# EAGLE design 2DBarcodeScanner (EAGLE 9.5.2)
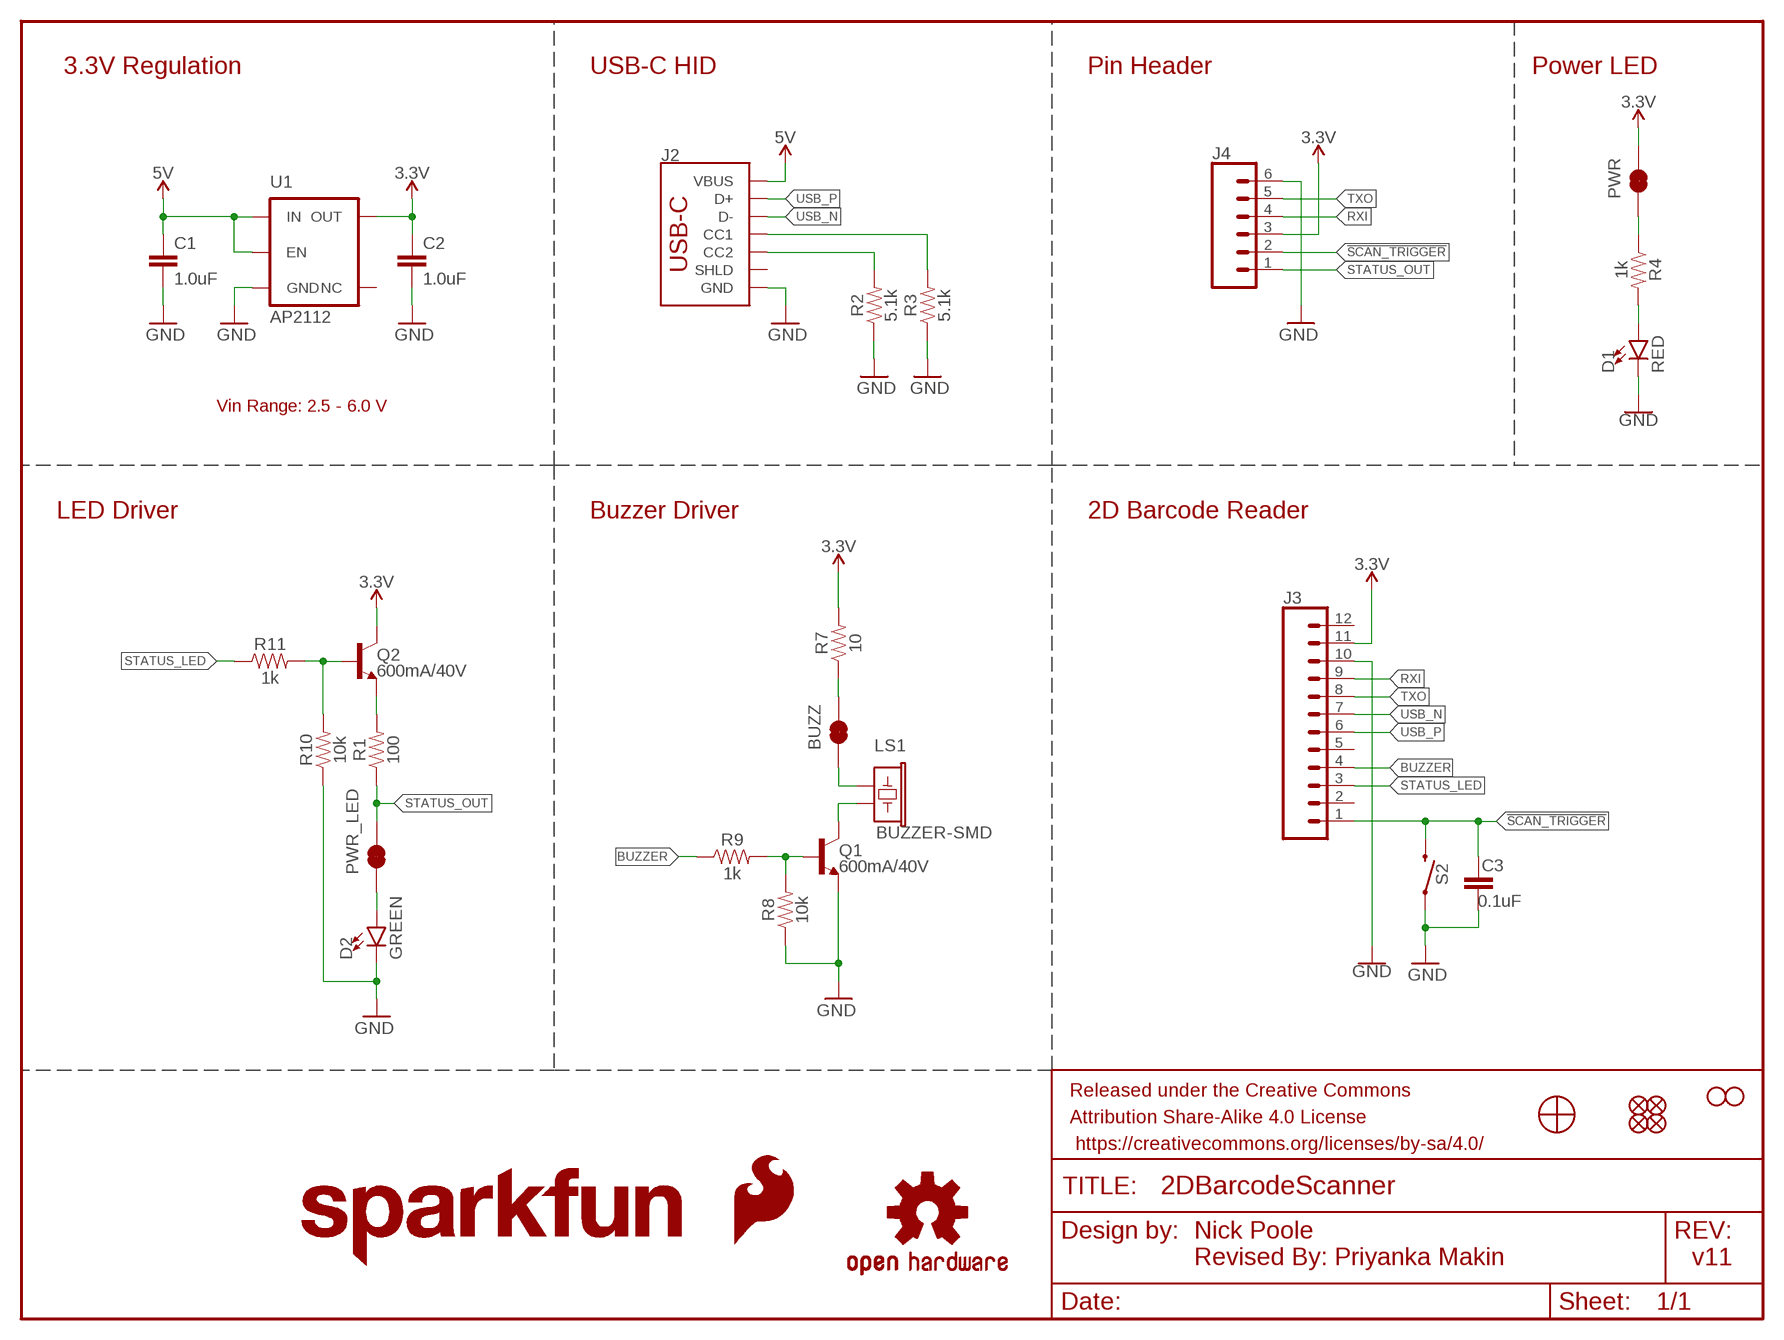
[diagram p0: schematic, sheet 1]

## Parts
BUZZ  JUMPER-SMT_2_NC_TRACE_SILK  [SMT-JUMPER_2_NC_TRACE_SILK]
C1  1.0uF  1.0UF-0603-16V-10%  [0603]
C2  1.0uF  1.0UF-0603-16V-10%  [0603]
C3  0.1uF  0.1UF-0603-25V-(+80/-20%)  [0603]
D1  RED  LED-RED0603  [LED-0603]
D2  GREEN  LED-GREEN0603  [LED-0603]
FD1  FIDUCIALUFIDUCIAL  [FIDUCIAL-MICRO]
FD2  FIDUCIALUFIDUCIAL  [FIDUCIAL-MICRO]
FD3  FIDUCIALUFIDUCIAL  [FIDUCIAL-MICRO]
FD4  FIDUCIALUFIDUCIAL  [FIDUCIAL-MICRO]
FRAME1  FRAME-LETTER  [CREATIVE_COMMONS]
H2  STAND-OFF  [STAND-OFF]
H3  STAND-OFF  [STAND-OFF]
J2  USB_C_2-LAYER_PADS  [USB-C-16P-2LAYER-PADS]
J3  CONN_12FPC_12_0.5MM  [FPC_12_0.5MM]
J4  CONN_06NO_SILK_FEMALE_PTH  [1X06_NO_SILK]
LOGO1  OSHW-LOGOS  [OSHW-LOGO-S]
LOGO2  SFE_LOGO_FLAME.1_INCH  [SFE_LOGO_FLAME_.1]
LOGO3  SFE_LOGO_NAME.1_INCH  [SFE_LOGO_NAME_.1]
LS1  BUZZER-SMD  [BUZZER-CCV]
PWR  JUMPER-SMT_2_NC_TRACE_SILK  [SMT-JUMPER_2_NC_TRACE_SILK]
PWR_LED  JUMPER-SMT_2_NC_TRACE_SILK  [SMT-JUMPER_2_NC_TRACE_SILK]
Q1  600mA/40V  TRANS_NPN-MMBT2222AL  [SOT23-3]
Q2  600mA/40V  TRANS_NPN-MMBT2222AL  [SOT23-3]
R1  100  100OHM-0603-1/10W-1%  [0603]
R2  5.1k  5.1KOHM5.1KOHM-0603-1/10W-1%  [0603]
R3  5.1k  5.1KOHM5.1KOHM-0603-1/10W-1%  [0603]
R4  1k  1KOHM-0603-1/10W-1%  [0603]
R7  10  10OHM-0603-1/10W-5%  [0603]
R8  10k  10KOHM-0603-1/10W-1%  [0603]
R9  1k  1KOHM-0603-1/10W-1%  [0603]
R10  10k  10KOHM-0603-1/10W-1%  [0603]
R11  1k  1KOHM-0603-1/10W-1%  [0603]
S2  MOMENTARY-SWITCH-SPST-SMD-5.2MM-TALL  [TACTILE_SWITCH_SMD_5.2MM]
U1  3.3V  V_REG_AP2112K-3.3V  [SOT23-5]
U2  BARCODE_SCANNER_MOUNT  [BARCODE_SCANNER_MOUNT]

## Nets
3.3V [power]: C2.1 J3.11 J4.3 PWR.2 Q2.3(C) R7.2 U1.5(OUT)
5V: C1.1 J2.VBUS1(VBUS) J2.VBUS2(VBUS) U1.1(IN) U1.3(EN)
!SCAN_TRIGGER!: C3.1 J3.1 J4.2 S2.3
BUZZER: J3.4 R9.1
CC3: J2.A5(CC1) R3.2
CC4: J2.B5(CC2) R2.2
GND [power]: C1.2 C2.2 C3.2 D1.C D2.C J2.GND J2.GND2(GND) J3.10 J4.6 Q1.2(E) R2.1 R3.1 R8.1 R10.1 S2.1 U1.2(GND)
N$1: BUZZ.2 R7.1
N$2: LS1.- Q1.3(C)
N$3: BUZZ.1 LS1.+
N$4: Q2.2(E) R1.2
N$5: Q1.1(B) R8.2 R9.2
N$6: PWR.1 R4.1
N$7: Q2.1(B) R10.2 R11.2
N$8: D2.A PWR_LED.1
N$9: D1.A R4.2
RXI: J3.9 J4.4
STATUS_LED: J3.3 R11.1
STATUS_OUT: J4.1 PWR_LED.2 R1.1
TXO: J3.8 J4.5
USB_N: J2.A7(D-) J2.B7(D-) J3.7
USB_P: J2.A6(D+) J2.B6(D+) J3.6
Unconnected: J2.SHLD1(SHLD) J2.SHLD2(SHLD) J2.SHLD3(SHLD) J2.SHLD4(SHLD) J3.2 J3.5 J3.12 U1.4(NC)

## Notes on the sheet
- 3.3V Regulation | USB-C HID | Pin Header | Power LED
- AP2112
- Vin Range: 2.5 - 6.0 V
- LED Driver | Buzzer Driver | 2D Barcode Reader
- Nick Poole
  Revised By: Priyanka Makin
- v11

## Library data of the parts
BUZZ PWR PWR_LED = SparkFun-Jumpers:JUMPER-SMT_2_NC_TRACE: Normally closed trace jumper
C1 C2 = SparkFun-Capacitors:1.0UF: 1µF ceramic capacitors; PROD_ID: CAP-00868
C3 = SparkFun-Capacitors:0.1UF: 0.1µF ceramic capacitors; PROD_ID: CAP-00810
D1 = SparkFun-LED:LED-RED: Red SMD LED; PROD_ID: DIO-00819
D2 = SparkFun-LED:LED-GREEN: Green SMD LED; PROD_ID: DIO-00821
FD1-FD4 = SparkFun-Aesthetics:FIDUCIAL: Fiducial Alignment Points
FRAME1 = SparkFun-Aesthetics:FRAME-LETTER: Schematic Frame - Letter
H2 H3 = SparkFun-Hardware:STAND-OFF: Stand Off
J2 = SparkFun-Connectors:USB_C: USB Type C 16Pin Connector Super Speed pins not available on the 16-pin purely SMD connector so this part is best for USB 2.0 implementations. D1 and D2 are tied together enabling D+/- no matter which way the cable is plugged into the connector. The two channel configuration pins (CC1/2) are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; PROD_ID: CONN-14122
J3 = SparkFun-Connectors:CONN_12: Multi connection point. Often used as Generic Header-pin footprint for 0.1 inch spaced/style header connections On any of the 0.1 inch spaced packages, you can populate with these: Break Away Headers - Straight (PRT-00116) Break Away Male Headers - Right Angle (PRT-00553) Female Headers (PRT-00115)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; PROD_ID: CONN-15766
J4 = SparkFun-Connectors:CONN_06: Multi connection point. Often used as Generic Header-pin footprint for 0.1 inch spaced/style header connections On any of the 0.1 inch spaced packages, you can populate with these: Break Away Headers - Straight (PRT-00116) Break Away Male Headers - Right Angle (PRT-00553) Female Headers (PRT-00115)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; PROD_ID: CONN-08437
LOGO1 = SparkFun-Aesthetics:OSHW-LOGO: Open-Source Hardware (OSHW) Logo
LOGO2 = SparkFun-Aesthetics:SFE_LOGO_FLAME: SparkFun Flame Logo
LOGO3 = SparkFun-Aesthetics:SFE_LOGO_NAME: SparkFun Font Logo
LS1 = SparkFun-Electromechanical:BUZZER: Buzzer; PROD_ID: COMP-08568
Q1 Q2 = SparkFun-DiscreteSemi:TRANS_NPN: NPN transistor Current controlled devices typically used to amplify current or used as a switch. BC547 - COM-08928 (TO-92 45V 100mA) (1.Collector 2.Base 3.Emitter) 2N3904 - COM-00521 (TO-92 40V 200mA) (1.Emitter 2.Base 3.Collector) P2N2222A - COM-12852 (TO-92 40V 600mA) (1.Collector 2.Base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; PROD_ID: TRANS-08049
R1 = SparkFun-Resistors:100OHM: 100Ω resistor; PROD_ID: RES-07863
R2 R3 = SparkFun-Resistors:5.1KOHM; PROD_ID: RES-12083
R4 R9 R11 = SparkFun-Resistors:1KOHM: 1kΩ resistor; PROD_ID: RES-07856
R7 = SparkFun-Resistors:10OHM: 10Ω resistor; PROD_ID: RES-09834
R8 R10 = SparkFun-Resistors:10KOHM: 10kΩ resistor; PROD_ID: RES-00824
S2 = SparkFun-Switches:MOMENTARY-SWITCH-SPST: Momentary Switch (Pushbutton) - SPST; PROD_ID: SWCH-14139
U1 = SparkFun-IC-Power:V_REG_AP2112: AP2112 - 600mA CMOS LDO Regulator w/ Enable The AP2112 is CMOS process low dropout linear regulator with enable function, the regulator delivers a guaranteed 600mA (min.) continuous load current. Features Output Voltage Accuracy: ±1.5% Output Current: 600mA (Min.) Foldback Short Current Protection: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; PROD_ID: VREG-12457
U2 = SparkFun-Hardware:BARCODE_SCANNER_MOUNT; PROD_ID: LPA-14926

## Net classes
1 power: width 0.178 mm

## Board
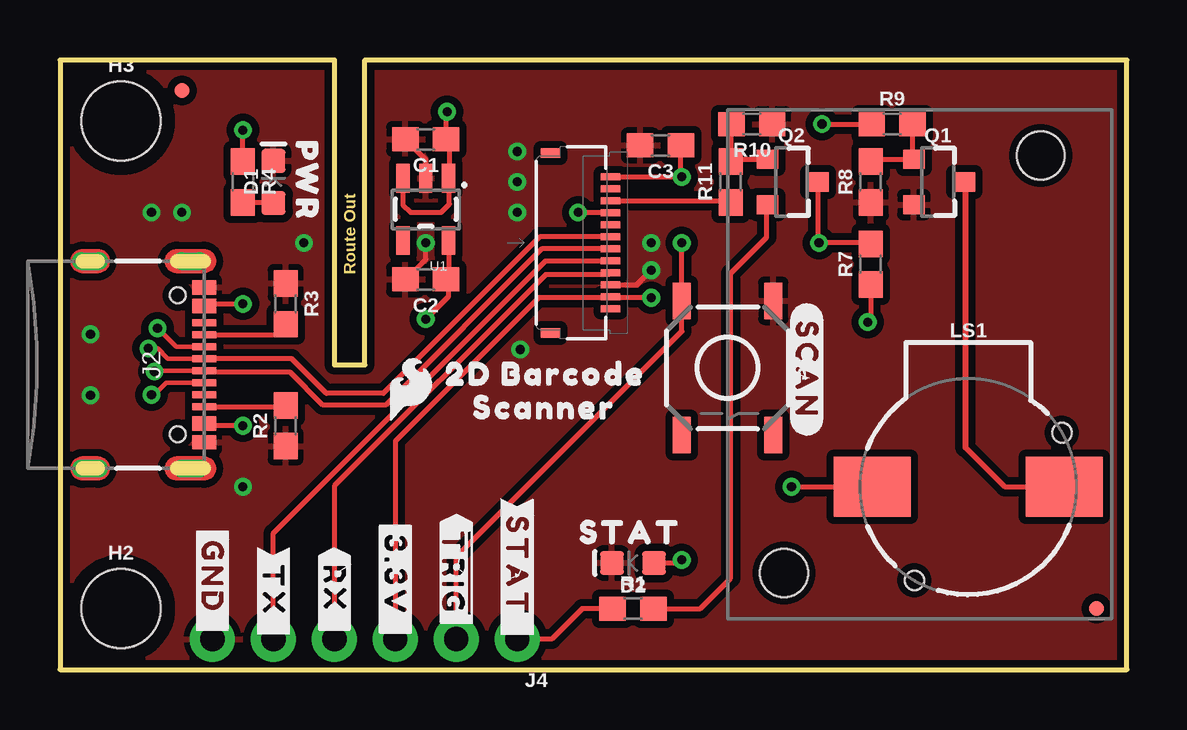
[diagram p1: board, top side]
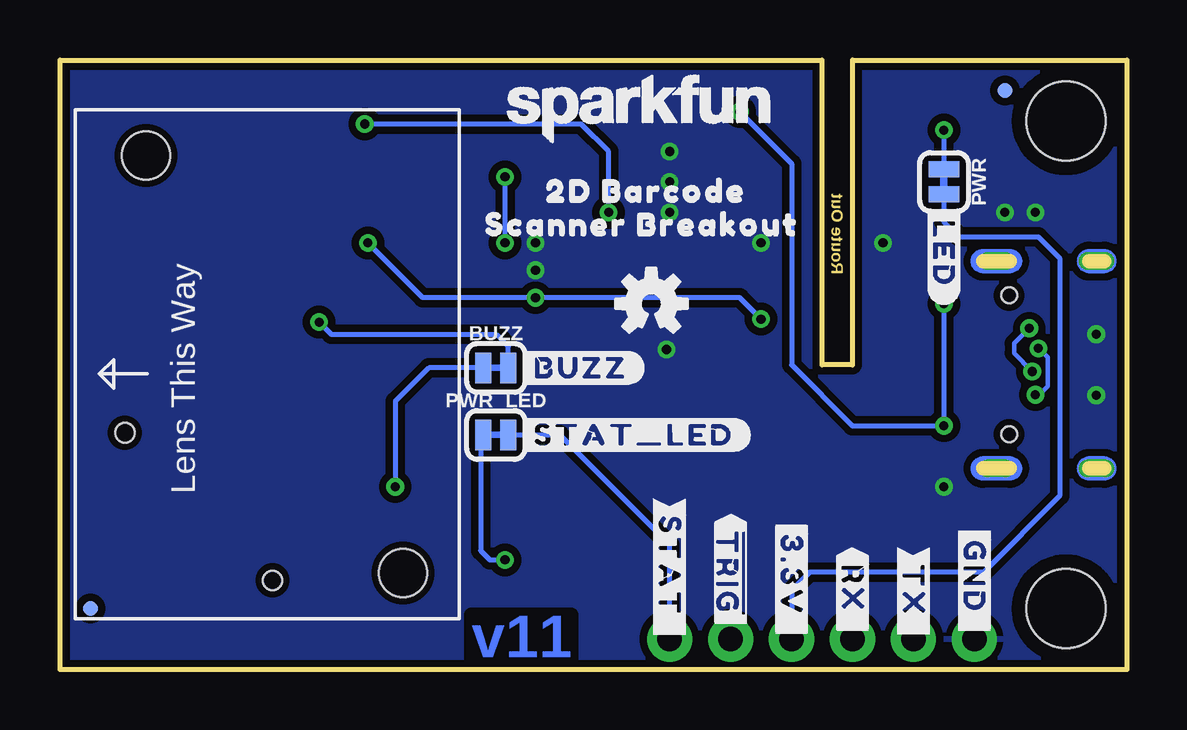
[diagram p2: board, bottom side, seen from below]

Size 44.45 x 25.4 mm. Coordinates in mm from the lower left corner, seen from the top.
Outline: 11.43,25.4 11.43,12.7 12.7,12.7 12.7,25.4 44.45,25.4 44.45,0 0,0 0,25.4 11.43,25.4
Copper layers (1*16): Top 0.035mm / dielectric 1.5mm / Bottom 0.035mm
Design rules "SparkFun-2-Layer-General-JLCPCB": minimum track width 7mil, minimum drill 0.3mm, track to track 7mil, track to pad 7mil, pad to pad 7mil, via to via 7mil, smd to smd 7mil, copper to edge 7mil, drill to drill 7mil, minimum pad ring 7mil, minimum via ring 7mil, stop-mask expansion 3mil, vias tented up to drill 25mil, thermal gap 10mil

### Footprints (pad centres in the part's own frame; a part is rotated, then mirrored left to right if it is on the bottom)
SMT-JUMPER_2_NC_TRACE_SILK = smd 0.66 x 1.27: 1 -0.521,0; 2 0.521,0
0603 = smd 1.1 x 1: 1 -0.85,0; 2 0.85,0
LED-0603 = smd 1 x 1: A -0.877,0; C 0.877,0
FIDUCIAL-MICRO = smd 0.635 x 0.635: 1 0,0
STAND-OFF = hole 3.302: 0,0
USB-C-16P-2LAYER-PADS = smd 0.3 x 1: A5 -1.25,-0.34; A6 -0.25,-0.34; A7 0.25,-0.34; A8 1.25,-0.34; B5 1.75,-0.34; B6 0.75,-0.34; B7 -0.75,-0.34; B8 -1.75,-0.34 | smd 0.6 x 1: GND -3.225,-0.34; GND2 3.225,-0.34; VBUS1 -2.45,-0.34; VBUS2 2.45,-0.34 | drill 0.4 pad 0.6 long: SHLD1 -4.318,-0.915; SHLD2 4.318,-0.915; SHLD3 -4.318,-5.095; SHLD4 4.318,-5.095 | hole 0.65: -2.89,-1.445; 2.89,-1.445
FPC_12_0.5MM = smd 0.3 x 0.8: 1 -2.75,1.35; 2 -2.25,1.35; 3 -1.75,1.35; 4 -1.25,1.35; 5 -0.75,1.35; 6 -0.25,1.35; 7 0.25,1.35; 8 0.75,1.35; 9 1.25,1.35; 10 1.75,1.35; 11 2.25,1.35; 12 2.75,1.35 | smd 0.4 x 0.8: MP1 -3.75,-1.15; MP2 3.75,-1.15
1X06_NO_SILK = drill 1.016 pad 1.88: 1 0,0; 2 2.54,0; 3 5.08,0; 4 7.62,0; 5 10.16,0; 6 12.7,0
BUZZER-CCV = smd 3.2 x 2.5: + 4,0; - -4,0 | hole 0.8: -3.9,-2.25; 2.25,3.9
SOT23-3 = smd 0.8 x 0.9: 1 -0.95,-1; 2 0.95,-1; 3 0,1.1
TACTILE_SWITCH_SMD_5.2MM = smd 1.524 x 0.762: 1 -2.794,1.905; 2 2.794,1.905; 3 -2.794,-1.905; 4 2.794,-1.905
SOT23-5 = smd 0.55 x 1.2: 1 -0.95,-1.3; 2 0,-1.3; 3 0.95,-1.3; 4 0.95,1.3; 5 -0.95,1.3
BARCODE_SCANNER_MOUNT = hole 2: -5.65,8.3; 5.05,-9.1

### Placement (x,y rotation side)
BUZZ  26.29,12.57 0 bottom
C1  15.24,22.1 180 top
C2  15.24,16.26 180 top
C3  25.02,21.84 180 top
D1  8.89,20.32 90 top
D2  23.88,4.45 180 top
FD1  5.08,24.13 0 top
FD2  43.18,2.54 0 top
FD3  43.18,2.54 0 bottom
FD4  5.08,24.13 0 bottom
FRAME1  not placed on the board
H2  2.54,2.54 0 top
H3  2.54,22.86 0 top
J2  6.35,12.7 270 top
J3  21.59,17.78 270 top
J4  19.05,1.27 180 top
LOGO1  19.81,15.24 0 bottom
LOGO2  14.61,11.68 0 top
LOGO3  20.32,23.37 0 bottom
LS1  37.85,7.62 180 top
PWR  7.62,20.32 270 bottom
PWR_LED  26.29,9.78 0 bottom
Q1  36.58,20.32 270 top
Q2  30.48,20.32 270 top
R1  23.88,2.54 0 top
R2  9.4,10.16 90 top
R3  9.4,15.24 270 top
R4  7.62,20.32 270 top
R7  33.78,16.89 90 top
R8  33.78,20.32 90 top
R9  34.67,22.73 0 top
R10  28.83,22.73 180 top
R11  27.94,20.32 90 top
S2  27.81,12.57 270 top
U1  15.24,19.18 180 top
U2  35.81,12.32 180 bottom
U$1  [##TRIG##0]  16.51,6.48 270 top
U$2  [#STAT_#0]  19.05,7.11 270 top
U$3  [STAT0]  20.95,5.71 0 top
U$4  [#SCAN#0]  31.11,15.24 270 top
U$5  [#BUZZ#0]  25.4,12.57 0 bottom
U$6  [#STAT_LED#0]  25.4,9.78 0 bottom
U$7  [##TRIG##0]  16.51,6.48 270 bottom
U$8  [PWR0]  10.29,22.73 270 top
U$9  [#LED#0]  7.62,19.43 270 bottom
U$17  [2D_BARCODE0]  15.37,12.32 0 top
U$18  [2D_BARCODE0]  24.89,19.94 0 bottom
U$19  [SCANNER0]  16.51,10.92 0 top
U$20  [SCANNER_BREAKOUT0]  27.43,18.54 0 bottom
U$21  [#STAT_#0]  19.05,7.11 270 bottom
U$26  [#TX_#0]  8.89,5.08 270 top
U$27  [#TX_#0]  8.89,5.08 270 bottom
U$28  [#3#3V_#0]  13.97,6.35 270 top
U$29  [#3#3V_#0]  13.97,6.35 270 bottom
U$30  [#RX_#0]  11.43,5.08 270 top
U$31  [#RX_#0]  11.43,5.08 270 bottom
U$32  [#GND_#0]  6.35,6.1 270 top
U$33  [#GND_#0]  6.35,6.1 270 bottom

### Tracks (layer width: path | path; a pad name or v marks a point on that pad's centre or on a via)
3.3V  (via drill 0.38)
  Top 0.203: J4.3 13.97,9.53 19.94,15.49 22.9,15.49 J3.11 22.98,15.49 v24.64,15.49 | R7.2 33.74,17.78 v31.62,17.78 31.58,17.82 Q2.3 | 16.19,16.36 C2.1 | U1.5 16.19,16.36 | 16.19,16.36 16.19,15.55 v15.24,14.61
  Bottom 0.203: v15.24,14.61 16.13,15.49 v24.64,15.49 29.34,15.49 v31.62,17.78 | PWR.2 7.62,18.67 6.99,18.03 3.68,18.03 2.79,17.14 2.79,7.24 5.97,4.06 13.21,4.06 13.97,3.3 J4.3
5V  (via drill 0.38)
  Top 0.178: 16.22,20.45 U1.1
  Top 0.203: J2.VBUS1 6.1,15.24 v7.62,15.24 | v7.62,10.16 6.1,10.16 J2.VBUS2 | v16.13,23.24 16.09,23.2 C1.1 16.22,21.97 16.22,20.45 16.22,19.39 15.88,19.05 14.61,19.05 14.29,19.36 U1.3
  Bottom 0.203: v7.62,15.24 v7.62,10.16 11.43,10.16 13.97,12.7 13.97,21.08 v16.13,23.24
!SCAN_TRIGGER!  (via drill 0.38)
  Top 0.203: v25.91,17.78 S2.3 25.91,14.1 16.51,4.7 J4.2 | C3.1 25.87,20.57 v25.91,20.53 J3.1
  Bottom 0.203: v25.91,17.78 v25.91,20.53
BUZZER  (via drill 0.38)
  Top 0.203: v31.75,22.73 R9.1 | J3.4 21.61,19.03 v21.59,19.05
  Bottom 0.203: v21.59,19.05 21.59,21.59 22.73,22.73 v31.75,22.73
CC3
  Top 0.178: J2.A5 6.29,13.95
  Top 0.203: 6.29,13.95 8.96,13.95 R3.2
CC4
  Top 0.203: J2.B5 9.34,10.95 R2.2
GND  (via drill 0.38)
  Top 0.203: C1.2 15.24,21.25 U1.2 | C2.2 15.24,17.11 v15.24,17.78 | J3.10 24.03,16.03 v24.64,16.64
  other vias: 5.08,19.05 3.81,19.05 10.16,17.78 1.27,13.97 1.27,11.43 19.18,13.34 24.64,17.78 19.05,21.59 19.05,20.32 19.05,19.05 7.62,7.62
  pour Top (isolate 0.305): 0,0 44.45,0 44.45,25.4 0,25.4
  pour Bottom (isolate 0.305): 0,25.4 0,0 44.45,0 44.45,25.4
N$1  (via drill 0.38)
  Top 0.203: R7.1 33.78,14.61 v33.66,14.48
  Bottom 0.203: v33.66,14.48 33.15,13.97 26.28,13.97 25.77,13.46 BUZZ.2
N$2
  Top 0.178: Q1.3 37.73,20.27
  Top 0.203: 37.73,9.26 39.37,7.62 LS1.-
  Top 0.254: 37.73,20.27 37.73,9.26
N$3  (via drill 0.38)
  Top 0.203: v30.48,7.62 LS1.+
  Bottom 0.203: BUZZ.1 29.08,12.57 30.48,11.18 v30.48,7.62
N$4
  Top 0.203: Q2.2 29.44,19.33 29.44,18.01 27.94,16.51 27.94,3.81 26.67,2.54 R1.2
N$5
  Top 0.203: R8.2 33.88,21.27 Q1.1 35.52,21.32 R9.2
N$6  (via drill 0.38)
  Top 0.203: R4.1 v7.62,22.48
  Bottom 0.203: v7.62,22.48 PWR.1
N$7
  Top 0.203: R10.2 27.98,21.21 R11.2 28.04,21.27 Q2.1
N$8  (via drill 0.38)
  Top 0.203: v25.91,4.57 25.78,4.45 D2.A
  Bottom 0.203: PWR_LED.1 26.92,9.66 26.92,4.95 26.54,4.57 v25.91,4.57
N$9
  Top 0.203: D1.A 7.65,19.44 R4.2
RXI
  Top 0.203: J3.9 22.87,16.46 20.24,16.46 11.43,7.65 J4.4
STATUS_LED
  Top 0.203: R11.1 27.88,19.53 J3.3
STATUS_OUT
  Top 0.203: R1.1 21.76,2.54 20.49,1.27 J4.1
  Bottom 0.203: PWR_LED.2 23.62,9.78 19.05,5.21 J4.1
TXO
  Top 0.203: J4.5 8.89,5.68 20.24,17.03 J3.8
USB_N  (via drill 0.38)
  Top 0.178: J2.B7 4.84,13.45 v4.06,14.22 | J2.A7 3.97,12.45 v3.94,12.42
  Top 0.203: J2.A7 6.07,12.39 9.59,12.39 10.96,11.02 13.56,11.02 20.07,17.53 J3.7
  Bottom 0.178: v4.06,14.22 4.7,13.59 4.7,13.18 v3.94,12.42
USB_P  (via drill 0.38)
  Top 0.178: J2.A6 4.5,12.95 4.06,13.39 v3.68,13.39 | J2.B6 4.43,11.95 3.94,11.46 v3.81,11.46
  Top 0.203: J2.A6 9.66,12.95 11.1,11.51 13.48,11.51 20,18.03 J3.6
  Bottom 0.178: v3.68,13.39 3.3,13.01 3.3,11.81 3.66,11.46 v3.81,11.46

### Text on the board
Bottom: v11
Dimension: Route Out
tDocu: Nick Poole / Revised by: Priyanka Makin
